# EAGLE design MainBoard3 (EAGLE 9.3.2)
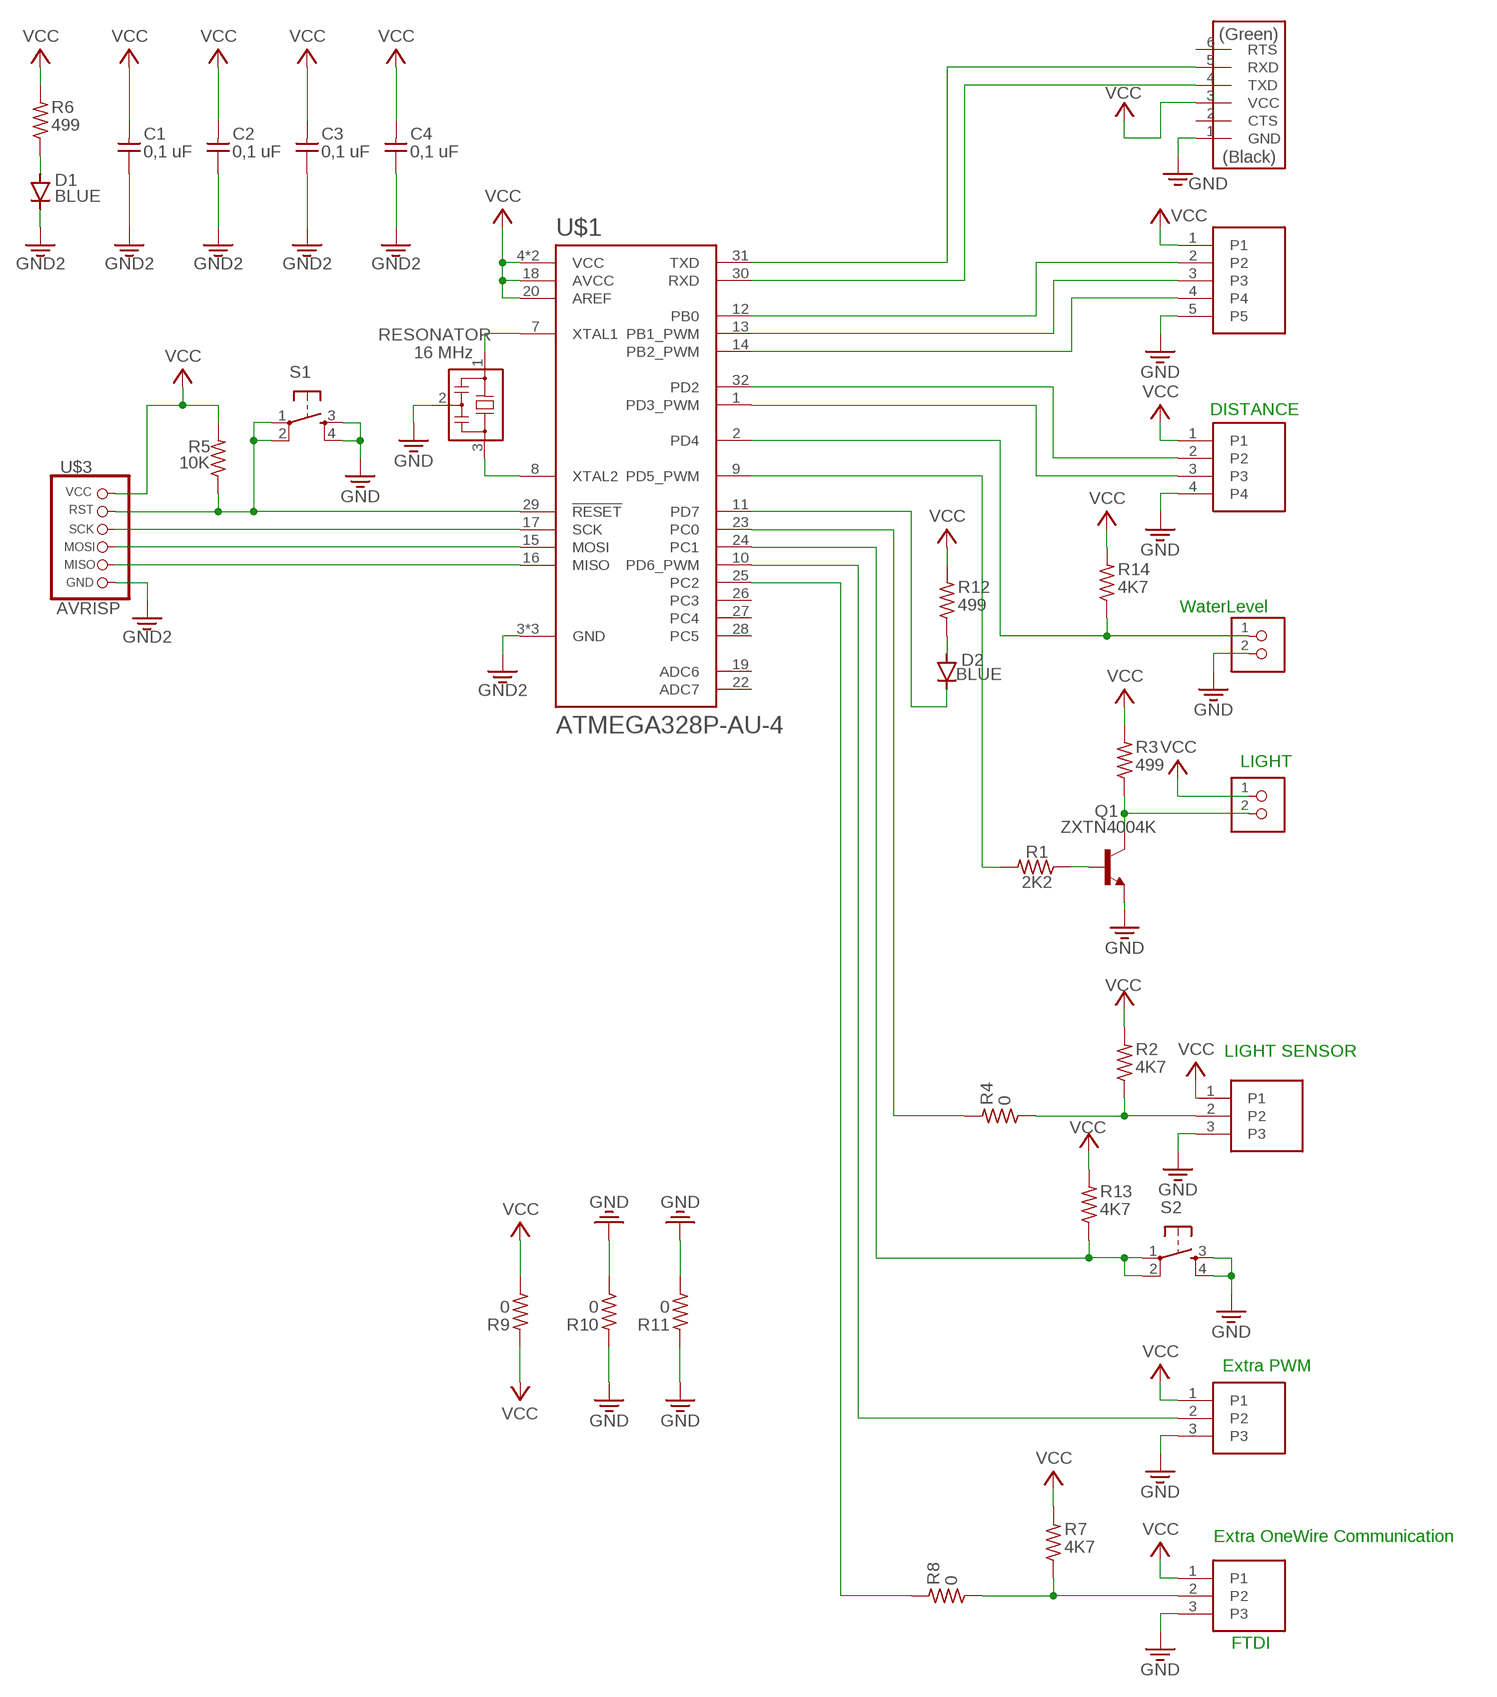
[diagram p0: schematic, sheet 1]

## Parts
C1  0,1 uF  CAP-UNPOLARIZED  [C1206]
C2  0,1 uF  CAP-UNPOLARIZED  [C1206]
C3  0,1 uF  CAP-UNPOLARIZED  [C1206]
C4  0,1 uF  CAP-UNPOLARIZED  [C1206]
D1  BLUE  CDBM1100-G  [MINI-SMA]
D2  BLUE  CDBM1100-G  [MINI-SMA]
LIGHT1  LIGHT  HEADERPIN_X3  [1X03SMD]
LIGHT2  LIGHT SENSOR  HEADERPIN_X3  [1X03SMD]
Q1  ZXTN4004K  [TO252]
R1  2K2  RES-US1206  [R1206]
R2  4K7  RES-US1206  [R1206]
R3  499  RES-US1206  [R1206]
R4  0  RES-US1206  [R1206]
R5  10K  RES-US1206  [R1206]
R6  499  RES-US1206  [R1206]
R7  4K7  RES-US1206  [R1206]
R8  0  RES-US1206  [R1206]
R9  0  RES-US1206  [R1206]
R10  0  RES-US1206  [R1206]
R11  0  RES-US1206  [R1206]
R12  499  RES-US1206  [R1206]
R13  4K7  RES-US1206  [R1206]
R14  4K7  RES-US1206  [R1206]
RESONATOR  16 MHz  RESONATOR  [EFOBM]
S1  6MM_SWITCH6MM_SWITCH  [6MM_SWITCH]
S2  6MM_SWITCH6MM_SWITCH  [6MM_SWITCH]
THERMO  THERMO  HEADERPIN_X3  [1X03SMD]
U$1  ATMEGA328P-AU-4  [QFP80P900X900X120-32N]
U$2  HEADERPIN_X5  [1X05SMD]
U$3  AVRISP  AVRISP_2SMD  [2X03SMD]
U$4  HEADERPIN_X2  [1X02SMD]
U$5  FTDI-SMD-HEADER  [1X06SMD]
U$6  HEADERPIN_X4  [1X04SMD]
U$7  HEADERPIN_X2  [1X02SMD]

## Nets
GND: C1.1 C2.1 C3.1 C4.1 D1.KATHODE LIGHT1.3 LIGHT2.3 Q1.2(E) R10.1 R10.2 R11.1 R11.2 RESONATOR.2 S1.3(S) S1.4(S1) S2.3(S) S2.4(S1) THERMO.3 U$1.3(GND) U$1.5(GND) U$1.21(GND) U$2.5 U$3.6(GND) U$5.1(GND) U$6.4 U$7.2 ; supply symbol labelled GND2
N$1: RESONATOR.1 U$1.7(XTAL1)
N$2: RESONATOR.3 U$1.8(XTAL2)
N$3: D1.ANODE R6.1
N$4: U$1.17(SCK) U$3.3(SCK)
N$5: U$1.15(MOSI) U$3.4(MOSI)
N$6: U$1.16(MISO) U$3.1(MISO)
N$7: U$1.12(PB0) U$2.2
N$8: U$1.13(PB1_PWM) U$2.3
N$9: U$1.14(PB2_PWM) U$2.4
N$10: R1.2 U$1.9(PD5_PWM)
N$11: LIGHT1.2 U$1.10(PD6_PWM)
N$12: R4.2 U$1.23(PC0)
N$13: R13.1 S2.1(P) S2.2(P1) U$1.24(PC1)
N$14: Q1.3(C) R3.1 U$4.2
N$15: Q1.1(B) R1.1
N$16: LIGHT2.2 R2.1 R4.1
N$17: R7.1 R8.1 THERMO.2
N$19: R5.1 S1.1(P) S1.2(P1) U$1.29(!RESET) U$3.5(RST)
N$20: R8.2 U$1.25(PC2)
N$21: D2.ANODE R12.1
N$23: D2.KATHODE U$1.11(PD7)
N$24: R14.1 U$1.2(PD4) U$7.1
N$26: U$1.32(PD2) U$6.2
N$27: U$1.1(PD3_PWM) U$6.3
N$28: U$1.30(RXD) U$5.4(TXD)
N$29: U$1.31(TXD) U$5.5(RXD)
VCC: C1.2 C2.2 C3.2 C4.2 LIGHT1.1 LIGHT2.1 R2.2 R3.2 R5.2 R6.2 R7.2 R9.1 R9.2 R12.2 R13.2 R14.2 THERMO.1 U$1.4(VCC) U$1.6(VCC) U$1.18(AVCC) U$1.20(AREF) U$2.1 U$3.2(VCC) U$4.1 U$5.3(VCC) U$6.1
Unconnected: U$1.19(ADC6) U$1.22(ADC7) U$1.26(PC3) U$1.27(PC4) U$1.28(PC5) U$5.2(CTS) U$5.6(RTS)

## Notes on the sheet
- DISTANCE
- WaterLevel
- LIGHT
- LIGHT SENSOR
- Extra PWM
- Extra OneWire Communication
- FTDI

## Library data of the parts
C1-C4 = Fablab:CAP-UNPOLARIZED
D1 D2 = Fablab:CDBM1100-G: Diode schottky 100V 1A mini-SMA as found in the fablab inventory
LIGHT1 LIGHT2 THERMO = Fablab:HEADERPIN_X3
Q1 = Fablab:ZXTN4004K: NPN Transistor
R1-R14 = Fablab:RES-US: Resistor (US Symbol)
RESONATOR = Fablab:RESONATOR
S1 S2 = Fablab:6MM_SWITCH: OMRON SWITCH
U$1 = ATMEGA328P-AU:ATMEGA328P-AU-4
U$2 = Fablab:HEADERPIN_X5
U$3 = Fablab:AVRISP_2
U$4 U$7 = Fablab:HEADERPIN_X2
U$5 = Fablab:FTDI-SMD-HEADER
U$6 = Fablab:HEADERPIN_X4

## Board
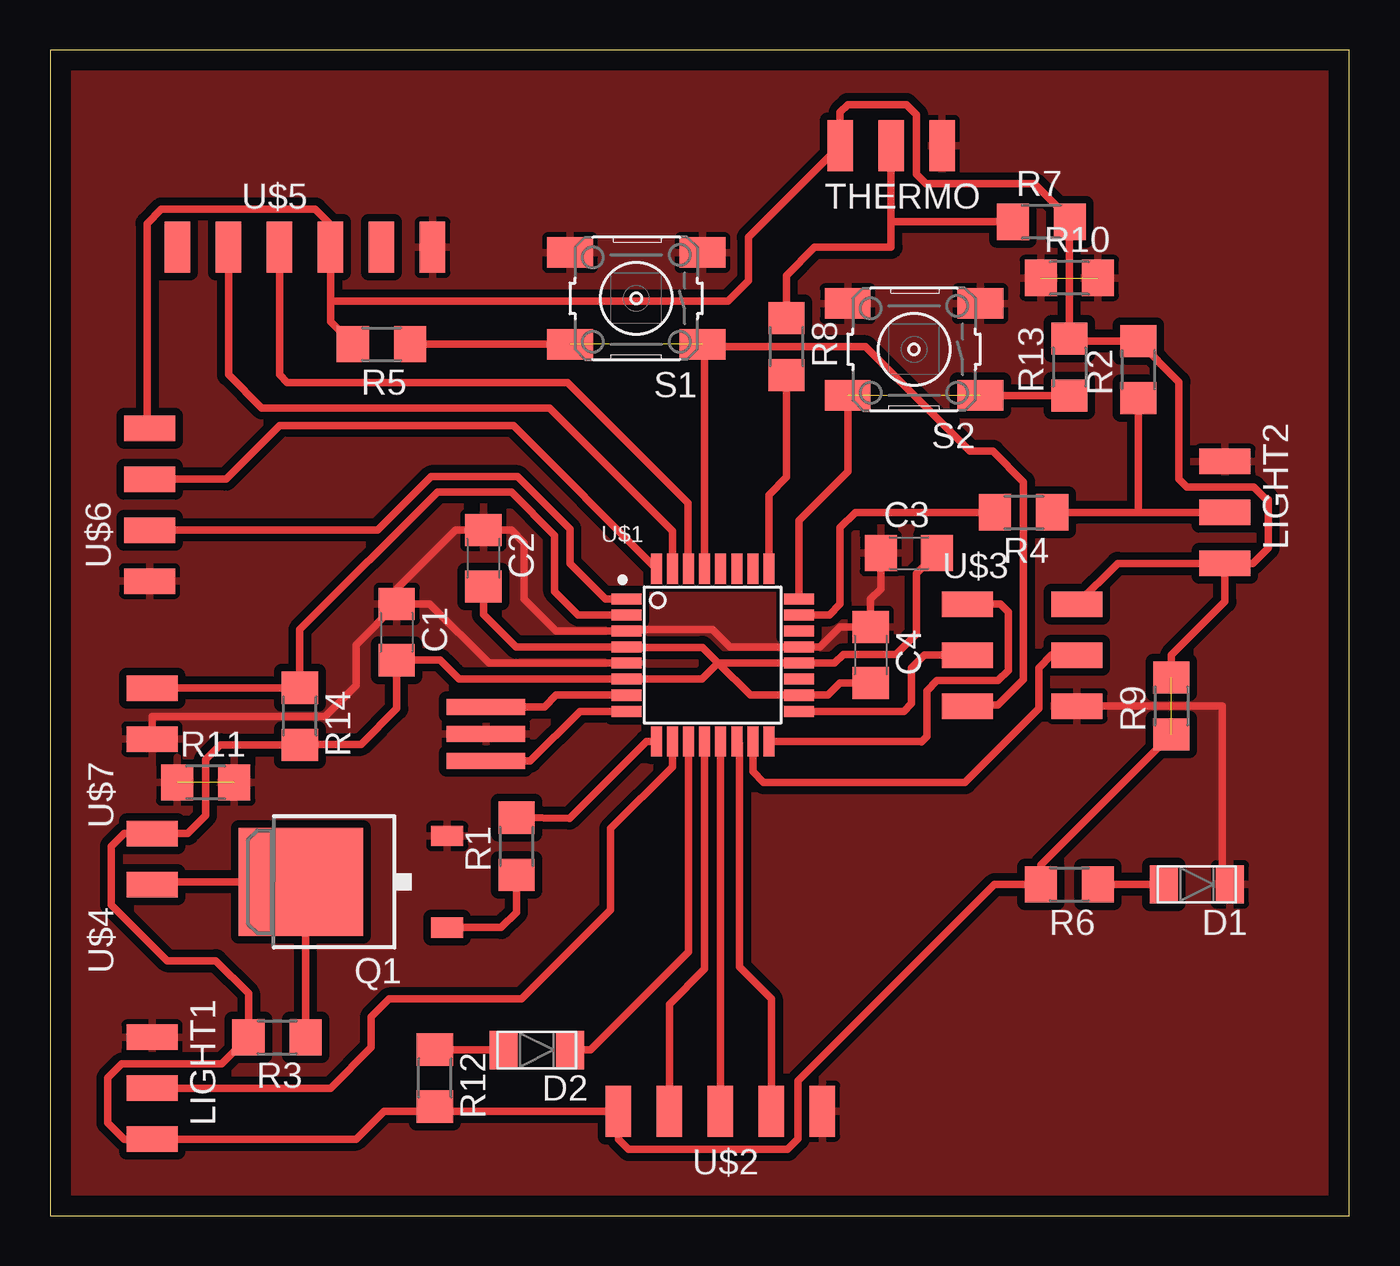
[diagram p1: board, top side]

Size 64.75 x 58.09 mm. Coordinates in mm from the lower left corner, seen from the top.
Outline: 0,0 64.75,0 64.75,58.09 0,58.09 0,0
Copper layers (1*16): Top 0.035mm / dielectric 1.5mm / Bottom 0.035mm
Design rules "default *": minimum track width 6mil, minimum drill 0.35mm, track to track 15mil, track to pad 15mil, pad to pad 15mil, via to via 15mil, smd to smd 6mil, copper to edge 40mil, drill to drill 6mil, minimum pad ring 10mil, minimum via ring 8mil, stop-mask expansion 4mil, vias tented up to drill 0mil, thermal gap 10mil

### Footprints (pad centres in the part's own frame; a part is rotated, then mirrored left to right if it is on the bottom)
C1206 = smd 1.6 x 1.8: 1 -1.4,0; 2 1.4,0
MINI-SMA = smd 1.4 x 1.9: ANODE 1.65,0; KATHODE -1.65,0
1X03SMD = smd 2.54 x 1.27: 1 0,3.81; 2 0,1.27; 3 0,-1.27
TO252 = smd 1 x 1.6: 1 -2.28,-6.07; 2 2.28,-6.07 | smd 5.4 x 6.2: 3 0,1.23
R1206 = smd 1.6 x 1.803: 1 -1.422,0; 2 1.422,0
EFOBM = smd 0.8 x 3.9: 1 -1.35,0; 2 0,0; 3 1.35,0
6MM_SWITCH = smd 2.286 x 1.524: 1 -3.302,2.286; 2 3.302,2.286; 3 -3.302,-2.286; 4 3.302,-2.286
QFP80P900X900X120-32N = smd 1.5 x 0.55: 1 -4.3,2.8; 2 -4.3,2; 3 -4.3,1.2; 4 -4.3,0.4; 5 -4.3,-0.4; 6 -4.3,-1.2; 7 -4.3,-2; 8 -4.3,-2.8; 17 4.3,-2.8; 18 4.3,-2; 19 4.3,-1.2; 20 4.3,-0.4; 21 4.3,0.4; 22 4.3,1.2; 23 4.3,2; 24 4.3,2.8 | smd 0.55 x 1.5: 9 -2.8,-4.3; 10 -2,-4.3; 11 -1.2,-4.3; 12 -0.4,-4.3; 13 0.4,-4.3; 14 1.2,-4.3; 15 2,-4.3; 16 2.8,-4.3; 25 2.8,4.3; 26 2,4.3; 27 1.2,4.3; 28 0.4,4.3; 29 -0.4,4.3; 30 -1.2,4.3; 31 -2,4.3; 32 -2.8,4.3
1X05SMD = smd 2.54 x 1.27: 1 0,3.81; 2 0,1.27; 3 0,-1.27; 4 0,-3.81; 5 0,-6.35
2X03SMD = smd 2.54 x 1.27: 1 -2.54,2.54; 2 2.92,2.54; 3 -2.54,0; 4 2.92,0; 5 -2.54,-2.54; 6 2.92,-2.54
1X02SMD = smd 2.54 x 1.27: 1 0,3.81; 2 0,1.27
1X06SMD = smd 2.54 x 1.27: 1 0,6.35; 2 0,3.81; 3 0,1.27; 4 0,-1.27; 5 0,-3.81; 6 0,-6.35
1X04SMD = smd 2.54 x 1.27: 1 0,3.81; 2 0,1.27; 3 0,-1.27; 4 0,-3.81

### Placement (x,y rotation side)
C1  17.27,29.08 270 top
C2  21.59,32.77 270 top
C3  42.8,33.02 0 top
C4  40.89,27.94 270 top
D1  57.15,16.51 180 top
D2  24.26,8.26 180 top
LIGHT1  5.08,7.62 180 top
LIGHT2  58.55,36.32 180 top
Q1  13.72,16.64 90 top
R1  23.24,18.41 90 top
R2  54.23,42.16 90 top
R3  11.3,8.89 180 top
R4  48.51,35.05 180 top
R5  16.51,43.43 180 top
R6  50.8,16.51 180 top
R7  49.4,49.53 0 top
R8  36.7,43.31 270 top
R9  55.88,25.4 90 top
R10  50.8,46.74 0 top
R11  7.75,21.59 0 top
R12  19.18,6.86 270 top
R13  50.8,42.29 90 top
R14  12.45,24.89 270 top
RESONATOR  21.72,24 270 top
S1  29.21,45.72 180 top
S2  43.05,43.18 180 top
THERMO  43.18,53.34 90 top
U$1  33.02,27.94 0 top
U$2  32.13,5.21 90 top
U$3  48.26,27.94 0 top
U$4  5.08,15.24 0 top
U$5  12.7,48.26 270 top
U$6  4.95,35.43 0 top
U$7  5.08,22.48 0 top

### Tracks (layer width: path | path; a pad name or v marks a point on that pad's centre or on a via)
GND  (2 unrouted)
  Top 0.381: C3.1 41.4,31.24 40.89,30.74 C4.1 39.37,29.34 38.37,28.34 U$1.21 33.89,28.34 33.02,29.21 28.79,29.21 U$1.3 25.22,29.14 23.62,30.73 23.62,33.53 22.98,34.17 C2.1 20.2,34.17 17.27,31.24 C1.1 | U$1.5 21.86,27.54 18.92,30.48 C1.1 | C1.1 15.24,28.45 15.24,26.42 13.72,24.89 5.08,24.89 U$7.2 | U$3.6 58.42,25.4 58.42,16.89 D1.KATHODE
  pour Top: 0,0 0,58.17 64.77,58.17 64.77,0
N$1
  Top 0.381: U$1.7 25.23,25.94 24.64,25.35 RESONATOR.1
N$2
  Top 0.381: U$1.8 26.41,25.14 23.92,22.65 RESONATOR.3
N$3
  Top 0.381: D1.ANODE R6.1
N$4
  Top 0.381: U$3.3 43.56,27.94 42.93,27.3 42.93,25.53 42.54,25.14 U$1.17
N$5
  Top 0.381: U$3.4 49.91,27.94 49.28,27.3 49.28,25.27 45.59,21.59 35.56,21.59 35.02,22.13 U$1.15
N$6
  Top 0.381: U$3.1 47.37,30.48 47.75,30.1 47.75,27.18 47.24,26.67 44.2,26.67 43.69,26.16 43.69,23.88 43.43,23.62 43.42,23.64 U$1.16
N$7
  Top 0.381: U$1.12 32.62,12.3 30.86,10.54 U$2.2
N$8
  Top 0.381: U$1.13 33.42,10.56 33.4,10.54 U$2.3
N$9
  Top 0.381: U$1.14 34.35,23.51 34.35,12.39 35.94,10.79 U$2.4
N$10
  Top 0.381: U$1.9 29.71,23.64 25.87,19.8 R1.2
N$11
  Top 0.381: LIGHT1.2 13.97,6.35 16,8.38 16,9.91 16.89,10.79 23.5,10.79 27.94,15.24 27.94,19.29 31.02,22.37 U$1.10
N$12
  Top 0.381: U$1.23 38.83,29.94 39.37,30.48 39.37,34.29 40.13,35.05 R4.2
N$13  (1 unrouted)
  Top 0.381: S2.2 39.75,37.08 37.32,34.65 U$1.24 | S2.1 46.38,40.87 R13.1
N$14
  Top 0.381: R3.1 12.72,16.4 Q1.3 5.21,16.64 U$4.2
N$15
  Top 0.381: Q1.1 22.48,14.36 23.24,15.11 R1.1
N$16
  Top 0.381: LIGHT2.2 54.23,35.05 | 54.23,35.05 R4.1 | R2.1 54.23,35.05
N$17
  Top 0.381: R8.1 36.7,46.86 38.1,48.26 41.91,48.26 41.91,49.53 | 41.91,49.53 THERMO.2 | R7.1 41.91,49.53
N$19  (1 unrouted)
  Top 0.381: U$3.5 45.78,25.46 47.24,25.46 48.51,26.73 48.51,36.58 46.99,38.1 45.85,38.1 40.64,43.31 32.64,43.31 S1.1 | 32.51,43.05 S1.1 | S1.2 R5.1 | S1.1 32.62,43.33 U$1.29
N$20
  Top 0.381: U$1.25 35.82,35.92 36.7,36.8 R8.2
N$21
  Top 0.381: D2.ANODE 19.2,8.26 R12.1
N$23
  Top 0.381: U$1.11 31.82,13.15 26.92,8.26 D2.KATHODE
N$24
  Top 0.381: U$1.2 26.32,29.94 25.15,31.11 25.15,33.91 22.99,36.07 19.3,36.07 12.45,29.21 R14.1 12.42,26.29 U$7.1
N$26
  Top 0.381: U$1.32 23.09,39.37 11.43,39.37 8.76,36.7 U$6.2
N$27
  Top 0.381: U$1.1 27.68,30.74 25.91,32.51 25.91,34.23 23.3,36.83 18.99,36.83 16.32,34.16 U$6.3
N$28
  Top 0.381: U$5.4 11.43,41.91 11.81,41.53 25.78,41.53 31.8,35.51 31.8,32.26 U$1.30
N$29
  Top 0.381: U$1.31 31.02,34.13 24.89,40.26 10.54,40.26 8.89,41.91 U$5.5
VCC  (1 unrouted)
  Top 0.381: 33.29,27.54 U$1.20 39.1,27.54 39.53,27.97 42.16,27.97 43.18,28.99 43.18,32 C3.2 | 33.29,27.54 32.51,28.32 28.74,28.32 U$1.4 23.22,28.34 21.59,29.97 C2.2 | 33.29,27.54 32.49,26.74 U$1.6 20.38,26.74 19.43,27.68 C1.2 17.27,25.27 15.49,23.5 12.47,23.5 R14.2 8.48,23.47 7.75,22.73 7.75,19.94 6.86,19.05 U$4.1 3.68,19.05 3.05,18.41 3.05,15.49 5.84,12.7 8.26,12.7 9.88,11.07 R3.2 8.55,7.56 3.57,7.56 2.88,6.86 2.88,4.62 3.68,3.81 LIGHT1.1 15.24,3.81 16.64,5.21 U$2.1 | 33.29,27.54 34.89,25.94 U$1.18 38.77,25.94 39.37,26.54 C4.2 | 13.97,45.59 U$5.3 13.97,49.4 13.21,50.16 5.54,50.16 4.83,49.45 4.83,39.37 U$6.1 | 13.97,45.59 13.97,44.55 R5.2 | R12.2 19.05,5.44 19.28,5.21 U$2.1 | U$2.1 28.32,3.81 28.83,3.3 36.75,3.3 37.27,3.83 37.27,6.71 47.07,16.51 R6.2 49.38,17.48 R9.1 | U$3.2 53.21,32.51 LIGHT2.1 | R9.2 55.88,27.94 58.55,30.61 LIGHT2.1 | LIGHT2.1 59.94,32.51 60.71,33.27 60.71,35.69 60.64,35.75 60.64,35.67 59.99,36.32 56.64,36.32 56.26,36.7 56.26,41.55 R2.2 50.93,43.59 R13.2 50.8,49.51 R7.2 50.83,49.66 49.05,51.44 43.64,51.44 43.18,51.9 43.18,54.86 42.67,55.37 39.75,55.37 39.37,54.99 THERMO.1 34.8,48.77 34.8,46.61 33.78,45.59 13.97,45.59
